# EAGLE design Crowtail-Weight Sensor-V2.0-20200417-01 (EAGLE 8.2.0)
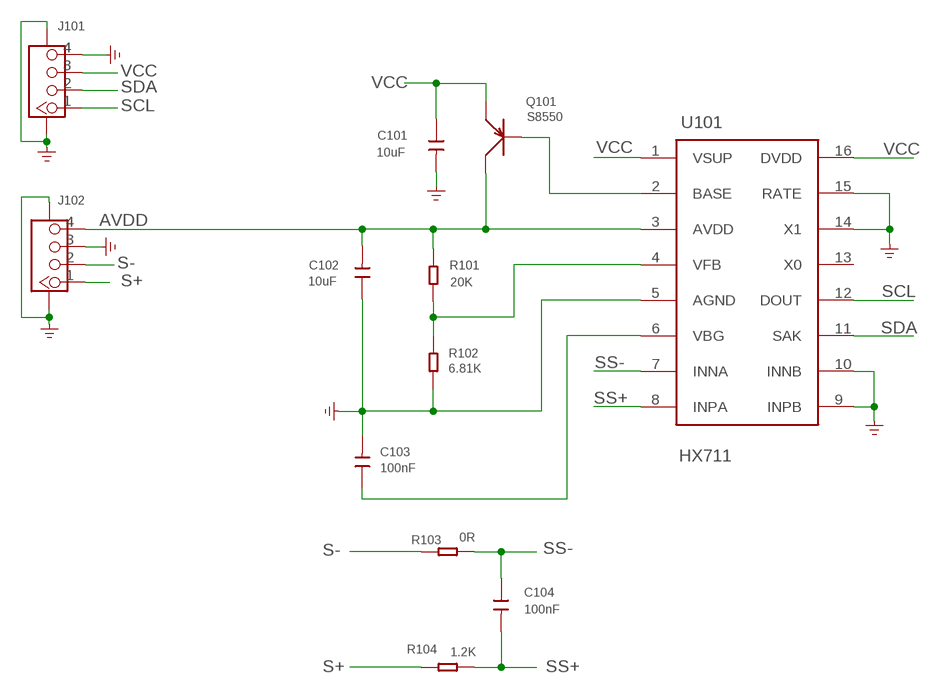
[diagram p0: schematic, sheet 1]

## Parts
C101  10uF  DISCRETE_C-0603  [DISCRETE_C0603]
C102  10uF  DISCRETE_C-0603  [DISCRETE_C0603]
C103  100nF  DISCRETE_C-0603  [DISCRETE_C0603]
C104  100nF  CAP-0603  [C0603]
J101  CONNECTOR_TWIG-4P-2.0-SMD-FEMALE-REINFORCE90D  [CONNECTOR_4P-SMD-2.0-90D]
J102  CONNECTOR_TWIG-4P-2.0-SMD-FEMALE-REINFORCE90D  [CONNECTOR_4P-SMD-2.0-90D]
Q101  S8550  TRANSISTOR-PNP-SOT23  [SOT23]
R101  20K  R-0603  [R0603]
R102  6.81K  R-0603  [R0603]
R103  0R  R-0603  [R0603]
R104  1.2K  R-0603  [R0603]
U101  HX711  IC_HX711  [IC_SOP16-L]

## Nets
AVDD: C102.2 J102.4 Q101.3(C) R101.2 U101.3(AVDD)
GND: C101.2 C102.1 C103.2 J101.4 J101.SS1 J101.SS2 J102.3 J102.SS1 J102.SS2 R102.1 U101.5(AGND) U101.9(INPB) U101.10(INNB) U101.14(X1) U101.15(RATE)
N$1: Q101.1(B) U101.2(BASE)
N$4: R101.1 R102.2 U101.4(VFB)
N$5: C103.1 U101.6(VBG)
S+: J102.1 R104.2
S-: J102.2 R103.1
SCL: J101.1 U101.12(DOUT)
SDA: J101.2 U101.11(SAK)
SS+: C104.2 R104.1 U101.8(INPA)
SS-: C104.1 R103.2 U101.7(INNA)
VCC: C101.1 J101.3 Q101.2(E) U101.1(VSUP) U101.16(DVDD)
Unconnected: U101.13(X0)

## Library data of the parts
C101-C103 = A_xbj:DISCRETE_C*: Ceramic Capacitors
C104 = Discrete-new:CAP: Ceramic Capacitors
J101 J102 = A_xbj:CONNECTOR_TWIG-4P-2.0-SMD-FEMALE-REINFORCE
Q101 = Discrete:TRANSISTOR-PNP*: PNP audion
R101-R104 = Discrete:R*
U101 = A_xbj:IC_HX711

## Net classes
0 default: width 0.305 mm, drill 0.305 mm, clearance 0.305 mm

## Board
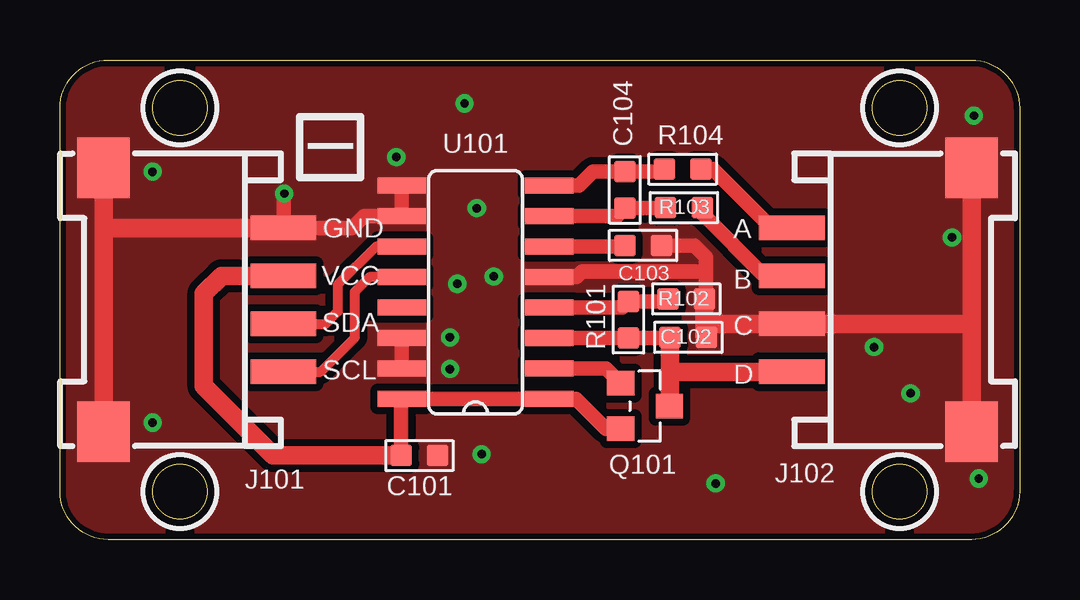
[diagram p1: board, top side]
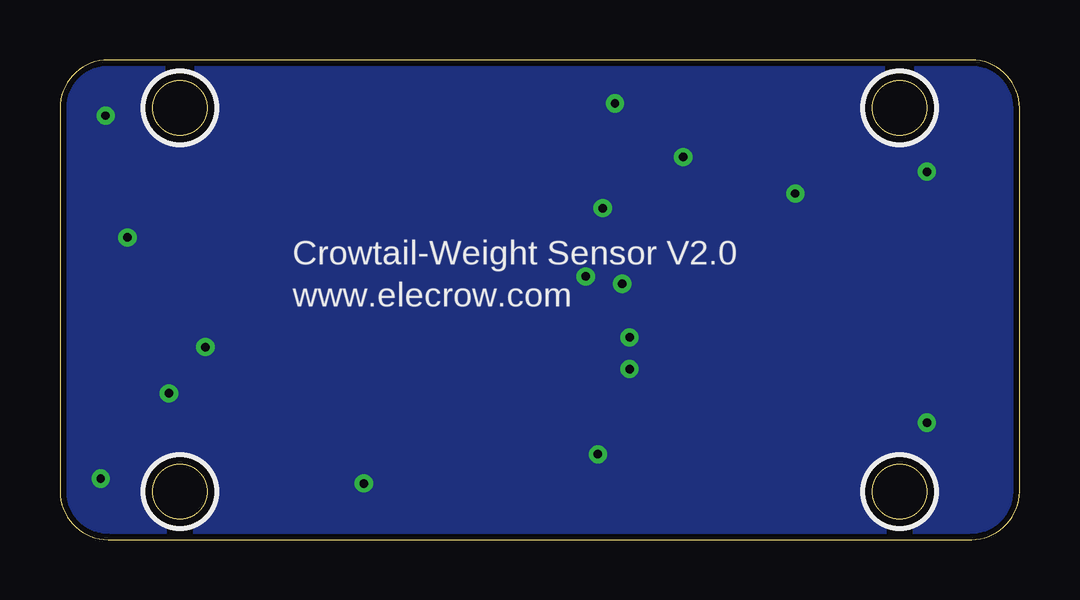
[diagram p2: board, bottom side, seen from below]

Size 40 x 20 mm. Coordinates in mm from the lower left corner, seen from the top.
Outline: 2,20 38,20 arc-90 40,18 40,2 arc-90 38,0 2,0 arc-90 0,2 0,18 arc-90 2,20
Outline: circle at 35,18 radius 1.14
Outline: circle at 35,2 radius 1.14
Outline: circle at 5,18 radius 1.14
Outline: circle at 5,2 radius 1.14
Copper layers (1*16): Top 0.035mm / dielectric 1.5mm / Bottom 0.035mm
Design rules "default": minimum track width 10mil, minimum drill 10mil, track to track 8mil, track to pad 8mil, pad to pad 8mil, via to via 8mil, smd to smd 8mil, copper to edge 10mil, drill to drill 8mil, minimum pad ring 10mil, minimum via ring 8mil, stop-mask expansion 4mil, vias tented up to drill 100mil, thermal gap 10mil
tRestrict: area 33.5,16.5 to 36.5,19.5; area 33.5,0.5 to 36.5,3.5; area 3.5,16.5 to 6.5,19.5; area 3.5,0.5 to 6.5,3.5
bRestrict: area 33.5,16.5 to 36.5,19.5; area 33.5,0.5 to 36.5,3.5; area 3.5,16.5 to 6.5,19.5; area 3.5,0.5 to 6.5,3.5

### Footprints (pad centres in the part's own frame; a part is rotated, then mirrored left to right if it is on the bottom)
DISCRETE_C0603 = smd 0.889 x 0.889: 1 -0.762,0; 2 0.762,0
C0603 = smd 0.889 x 0.889: 1 0,0.762; 2 0,-0.762
CONNECTOR_4P-SMD-2.0-90D = smd 1.01 x 2.74: 1 -3,-0.1; 2 -1,-0.1; 3 1,-0.1; 4 3,-0.1 | smd 2.54 x 2.184: SS1 -5.5,7.4; SS2 5.5,7.4
SOT23 = smd 1.016 x 1.143: 1 -0.95,-1.016; 2 0.95,-1.016; 3 0,1.016
R0603 = smd 0.889 x 0.889: 1 -0.762,0; 2 0.762,0
IC_SOP16-L = smd 0.66 x 2.032: 1 -4.445,-3.073; 2 -3.175,-3.073; 3 -1.905,-3.073; 4 -0.635,-3.073; 5 0.635,-3.073; 6 1.905,-3.073; 7 3.175,-3.073; 8 4.445,-3.073; 9 4.445,3.073; 10 3.175,3.073; 11 1.905,3.073; 12 0.635,3.073; 13 -0.635,3.073; 14 -1.905,3.073; 15 -3.175,3.073; 16 -4.445,3.073

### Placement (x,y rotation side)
C101  14.98,3.5 0 top
C102  26.19,8.43 180 top
C103  24.31,12.27 0 top
C104  23.55,14.58 180 top
J101  9.22,10 90 top
J102  30.61,10 270 top
Q101  24.39,5.57 270 top
R101  23.7,9.17 270 top
R102  26.11,10.03 180 top
R103  26.01,13.84 180 top
R104  25.96,15.44 0 top
U101  17.32,10.31 90 top

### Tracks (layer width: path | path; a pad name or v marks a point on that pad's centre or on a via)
AVDD
  Top 0.61: U101.3 R101.2 25.41,8.41 C102.2
  Top 0.762: 25.43,6.91 C102.2 | 25.43,6.91 25.43,5.59 Q101.3 | J102.4 25.52,7 25.43,6.91
GND  (via drill 0.35)
  Top 0.406: 29.83,9 J102.3
  Top 0.61: C103.2 26.44,12.27 26.92,11.79 26.92,11.18 | 26.92,10.08 26.92,11.18 | 26.92,10.08 R102.1 | 26.95,10.05 26.92,10.08 | U101.9 U101.10 12.68,13.49 12.19,13 J101.4 9.31,14.39 v9.35,14.43 | U101.14 U101.15 | 26.92,11.18 21.77,11.18 21.54,10.95 U101.5
  Top 0.762: 1.81,13.01 J101.SS1 | 1.81,13.01 J101.SS2 | J101.4 1.82,13 1.81,13.01 | 26.87,8.94 R102.1 | 26.87,8.94 26.87,8.51 C102.1 | 26.87,8.94 26.93,9 J102.3 37.97,9 38.01,9.04 | 38.01,9.04 J102.SS1 | 38.01,9.04 J102.SS2
  other vias: 17.37,13.82 16.87,18.19 16.56,10.67 17.58,3.56 3.86,4.88 3.86,15.34 14.02,15.95 38.1,17.68 38.3,2.54 33.93,8.03 18.08,10.97 16.26,8.43 16.26,7.11 37.19,12.6 35.46,6.1 27.33,2.34
  pour Top (no thermals): 40.76,2.79 40.76,18.29 arc90 38.48,20.57 1.65,20.57 arc90 -0.64,18.29 -0.64,2.03 arc90 2.15,-0.76 37.21,-0.76 arc90
  pour Bottom (no thermals): 40.76,2.79 40.76,18.57 arc90 38.76,20.57 1.14,20.57 arc90 -0.64,18.8 -0.64,2.03 arc90 2.15,-1.27 37.21,-1.27 arc90
N$1
  Top 0.61: U101.2 22.75,7.14 Q101.1
N$4
  Top 0.61: U101.4 23.44,9.68 R101.1 25.25,9.93 R102.2
N$5
  Top 0.61: U101.6 23.5,12.22 C103.1
S+
  Top 0.61: R104.2 27.23,15.44 29.67,13 J102.1
S-
  Top 0.61: J102.2 29.36,11 26.77,13.59 R103.1
SCL
  Top 0.406: U101.12 12.9,10.95 12.29,10.34 12.29,8.43 10.86,7 J101.1
SDA
  Top 0.406: U101.11 13.17,12.22 11.58,10.63 11.58,9.51 11.07,9 J101.2
SS+
  Top 0.61: R104.1 25.09,15.34 C104.2 22.23,15.34 21.64,14.76 U101.8
SS-
  Top 0.61: R103.2 25.22,13.82 C104.1 23.22,13.49 U101.7
VCC
  Top 0.61: C101.1 14.22,5.84 U101.16 U101.1 21.51,5.87 22.76,4.62 Q101.2
  Top 0.762: J101.3 6.73,11 5.99,10.26 5.99,6.4 8.89,3.5 C101.1

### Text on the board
tPlace: I | GND | A | VCC | B | SDA | C | SCL | D
bPlace: Crowtail-Weight Sensor V2.0 | www.elecrow.com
